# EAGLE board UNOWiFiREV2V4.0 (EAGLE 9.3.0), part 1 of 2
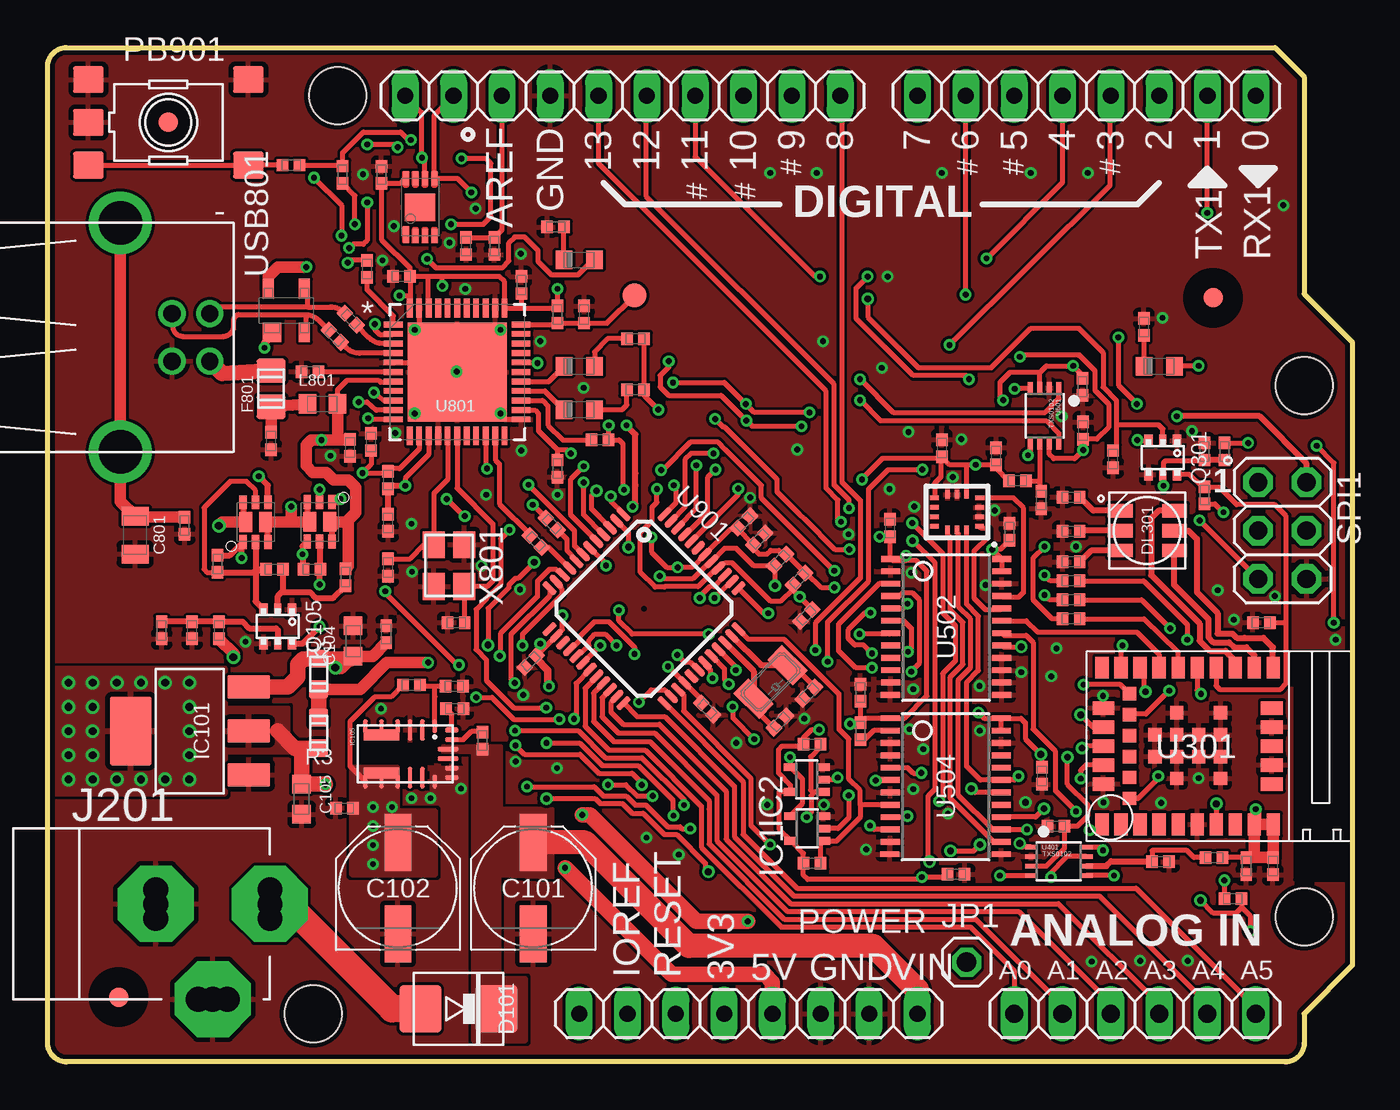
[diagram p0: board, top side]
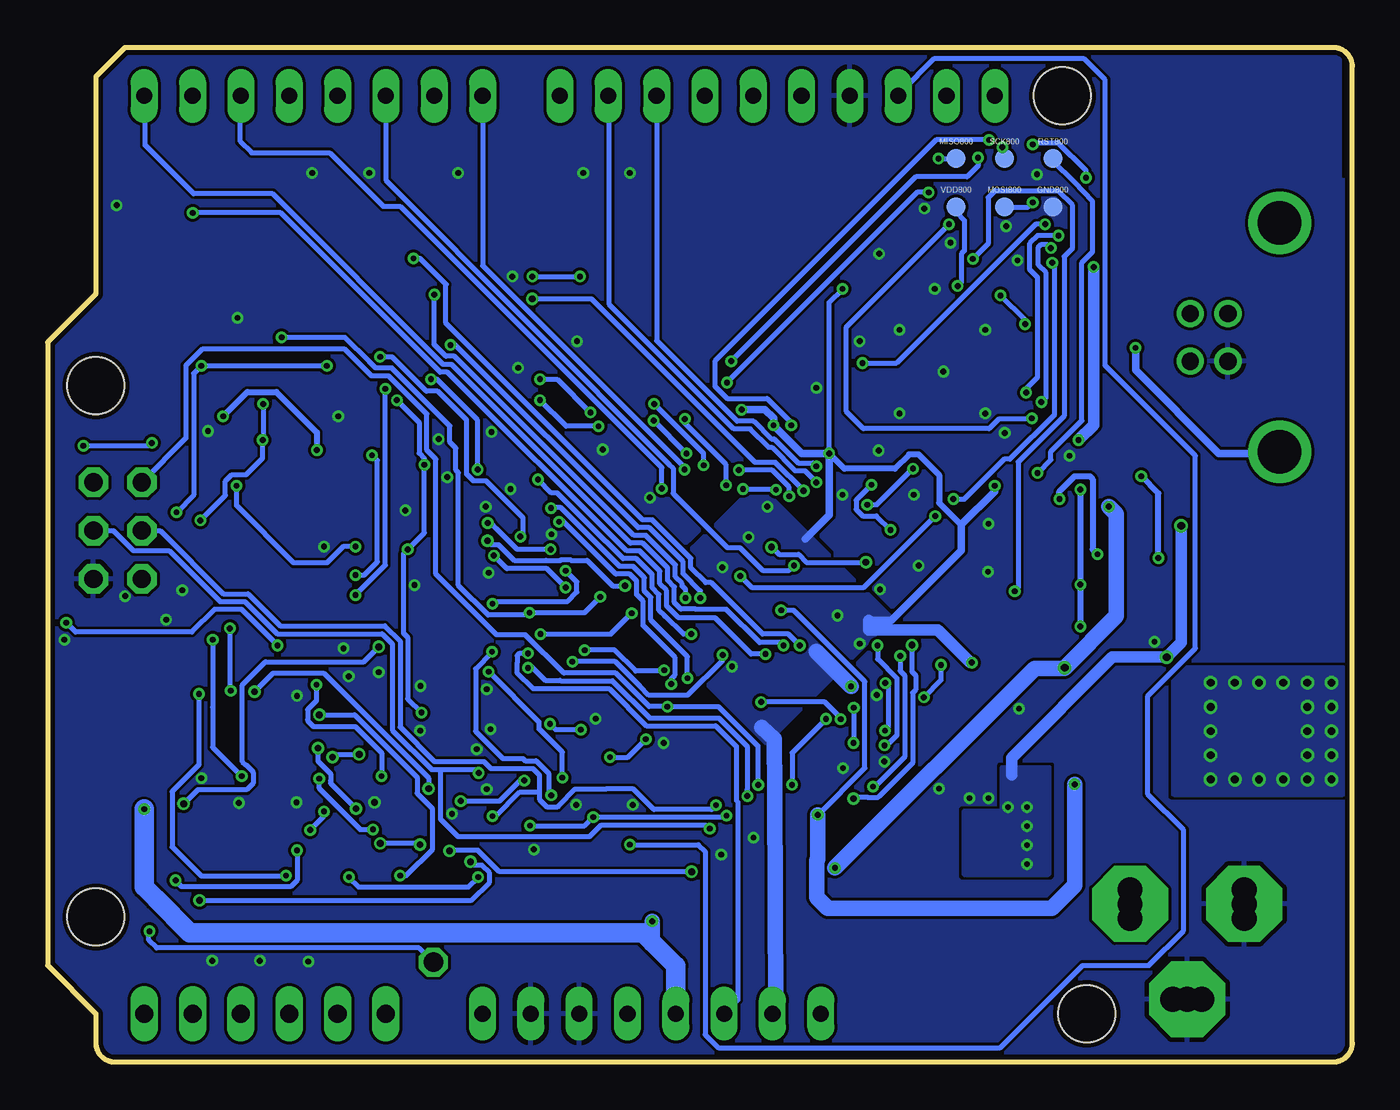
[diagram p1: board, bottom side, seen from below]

Size 68.58 x 53.34 mm. Coordinates in mm from the lower left corner, seen from the top.
Outline: 64.52,53.34 66.04,51.82 66.04,40.39 68.58,37.85 68.58,5.08 66.04,2.54 66.04,1 arc-90 65.04,0 1,0 arc-90 0,1 0,52.34 arc-90 1,53.34 64.52,53.34
Copper layers (1*16): Top 0.035mm / dielectric 1.5mm / Bottom 0.035mm
Design rules "SeeedStudio_2layers": minimum track width 6mil, minimum drill 12mil, track to track 6mil, track to pad 6mil, pad to pad 6mil, via to via 6mil, smd to smd 0mil, copper to edge 10mil, drill to drill 10mil, minimum pad ring 10mil, minimum via ring 6mil, stop-mask expansion 2mil, vias tented up to drill 100mil, thermal gap 10mil
Net classes: 0 default: width 0.006 mm, drill 0.305 mm
Holes 3 mm at 66.04,35.56 66.04,7.62 15.24,50.8 13.97,2.54
tRestrict: 3 lines

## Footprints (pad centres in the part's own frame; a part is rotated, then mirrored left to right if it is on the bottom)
1X06-TH = drill 0.95 pad 1.422 long: 1 -6.35,0; 2 -3.81,0; 3 -1.27,0; 4 1.27,0; 5 3.81,0; 6 6.35,0
0402-1005X55N = smd 0.62 x 0.62: 1 -0.45,0; 2 0.45,0
PANASONIC_D = smd 3 x 1.4: + 2.4,0; - -2.4,0
0603-1608X90N = smd 0.95 x 1: 1 -0.8,0; 2 0.8,0
0805-R2013X50N = smd 0.95 x 1.45: 1 -1,0; 2 1,0
SMB_DO214AA = smd 2.2 x 2.5: A -2,0; C 2,0
SOT190P230X110-4N = smd 1 x 1: 1 -1.15,0.75 | smd 1 x 0.6: 2 -1.15,-0.95; 3 1.15,-0.95; 4 1.15,0.95
RGBLED = smd 1.3 x 0.7: 1 -1.425,1.05; 2 -1.425,0; 3 -1.425,-1.05; 4 1.425,-1.05; 5 1.425,0; 6 1.425,1.05
C0805 = smd 1.25 x 1.5: 1 -0.95,0; 2 0.95,0
FD-1-2 = smd 1.016 x 1.016: P$1 0,0
TP-1.00MM = smd 1 x 1 bottom: X 0,0
SC70-5 = smd 0.4 x 0.7: 1 -0.65,-0.85; 2 0,-0.85; 3 0.65,-0.85; 4 0.65,0.85; 5 -0.65,0.85
SOT223 = smd 2.235 x 1.219: 1 -3.099,2.311; 2 -3.099,0; 3 -3.099,-2.311 | smd 2.2 x 3.6: 4 3.099,0
MPM3610 = smd 0.7 x 0.25: 1 -1.45,1.55; 4 -1.45,-0.4; 5 -1.45,-1.25; 6 -1.45,-2.1; 7 1.45,-2.1; 8 1.45,-1.25; 9 1.45,-0.4; 12 1.45,1.55 | smd 1.1 x 0.25: 2 -1.25,0.9; 3 -1.25,0.25; 10 1.25,0.25; 11 1.25,0.9 | smd 0.25 x 0.7: 13 1.25,2.45; 14 0.75,2.45; 17 -0.75,2.45; 18 -1.25,2.45 | smd 0.25 x 1.1: 15 0.25,2.25; 16 -0.25,2.25 | smd 0.6 x 1.95: 19 -1,-1.25; 20 1,-1.25
1X10 = drill 0.85 pad 1.422 long: 1 -11.43,0; 2 -8.89,0; 3 -6.35,0; 4 -3.81,0; 5 -1.27,0; 6 1.27,0; 7 3.81,0; 8 6.35,0; 9 8.89,0; 10 11.43,0
1X08 = drill 0.85 pad 1.422 long: 1 -8.89,0; 2 -6.35,0; 3 -3.81,0; 4 -1.27,0; 5 1.27,0; 6 3.81,0; 7 6.35,0; 8 8.89,0
POWERSUPPLY_DC-21MM = drill 1.3 pad 4 octagon: +1 -0.076,-6.35; -1 -0.076,-0.356; E1 -5.08,-3.353 | drill 1.3: +2 -0.838,-6.35; +3 0.686,-6.35; -2 -0.838,-0.356; -3 0.686,-0.356; E2 -5.08,-2.591; E3 -5.08,-4.115
1X01 = drill 1.016 octagon: 1 0,0
LEDC1608X80N-AK = smd 0.9 x 0.95: A 0.8,0; C -0.8,0
TS42 = smd 1.6 x 1.4: 1 4.2,-2.25; 2 -4.2,-2.25; 3 4.2,2.25; 4 -4.2,2.25; 5 4.2,0
PWR_SC70 = smd 0.4 x 0.69: D1 -0.65,1.04; D2 0.65,-1.04; G1 0,-1.04; G2 0,1.04; S1 -0.65,-1.04; S2 0.65,1.04 | smd 0.7 x 1: D1' -0.525,0; D2' 0.525,0
SOT363 = smd 0.5 x 0.6: 1 -0.75,-0.9; 3 0.75,-0.9; 4 0.75,0.9; 6 -0.75,0.9 | smd 0.4 x 0.6: 2 0,-0.9; 5 0,0.9
C0603 = smd 0.95 x 1: 1 -0.8,0; 2 0.8,0
2X03 = drill 0.95 pad 1.55 octagon: 1 2.54,1.27; 2 2.54,-1.27; 3 0,1.27; 4 0,-1.27; 5 -2.54,1.27; 6 -2.54,-1.27
TP-1.27MM = smd 1.27 x 1.27 bottom: X 0,0
LGA14L = smd 0.45 x 0.25: 1 -1.175,0.75; 2 -1.175,0.25; 3 -1.175,-0.25; 4 -1.175,-0.75; 8 1.175,-0.75; 9 1.175,-0.25; 10 1.175,0.25; 11 1.175,0.75 | smd 0.25 x 0.45: 5 -0.5,-0.925; 6 0,-0.925; 7 0.5,-0.925; 12 0.5,0.925; 13 0,0.925; 14 -0.5,0.925
NINA-W1X = smd 0.7 x 1.15: 1 4.95,4.125; 2 3.95,4.125; 3 2.95,4.125; 4 1.95,4.125; 5 0.95,4.125; 6 -0.05,4.125; 7 -1.05,4.125; 8 -2.05,4.125; 9 -3.05,4.125; 10 -4.05,4.125; 16 -4.05,-4.125; 17 -3.05,-4.125; 18 -2.05,-4.125; 19 -1.05,-4.125; 20 -0.05,-4.125; 21 0.95,-4.125; 22 1.95,-4.125; 23 2.95,-4.125; 24 3.95,-4.125; 25 4.95,-4.125 | smd 1.15 x 0.7: 11 -3.975,2; 12 -3.975,1; 13 -3.975,0; 14 -3.975,-1; 15 -3.975,-2; 26 4.875,-2; 27 4.875,-1; 28 4.875,0; 29 4.875,1; 30 4.875,2 | smd 0.7 x 0.7: 31 3.5,2.75; 32 3.5,1.65; 33 3.5,0.55; 34 3.5,-0.55; 35 3.5,-1.65; 36 3.5,-2.75; GND@1 -1.28,1.7; GND@2 -1.28,0.55; GND@3 -1.28,-0.6; GND@4 -1.28,-1.75; GND@5 -0.13,0.55; GND@6 -0.13,-0.6; GND@7 1.02,1.7; GND@8 1.02,0.55; GND@9 1.02,-0.6; GND@10 1.02,-1.75; GND@11 2.17,0.55; GND@12 2.17,-0.6
VFSOP-8 = smd 0.25 x 0.65: P$1 -0.75,-1.45; P$2 -0.25,-1.45; P$3 0.25,-1.45; P$4 0.75,-1.45; P$5 0.75,1.45; P$6 0.25,1.45; P$7 -0.25,1.45; P$8 -0.75,1.45
TSSOP24 = smd 0.305 x 0.991: 1 -3.575,-2.918; 2 -2.925,-2.918; 3 -2.275,-2.918; 4 -1.625,-2.918; 5 -0.975,-2.918; 6 -0.325,-2.918; 7 0.325,-2.918; 8 0.975,-2.918; 9 1.625,-2.918; 10 2.275,-2.918; 11 2.925,-2.918; 12 3.575,-2.932; 13 3.575,2.918; 14 2.925,2.918; 15 2.275,2.918; 16 1.625,2.918; 17 0.975,2.918; 18 0.325,2.918; 19 -0.325,2.918; 20 -0.975,2.918; 21 -1.625,2.918; 22 -2.275,2.918; 23 -2.925,2.918; 24 -3.575,2.918
SON50P300X200X60-9N-EP160X140 = smd 0.3 x 0.85: 1 -0.75,-1.45 | smd 0.3 x 0.7: 2 -0.25,-1.525; 3 0.25,-1.525; 4 0.75,-1.525; 5 0.75,1.525; 6 0.25,1.525; 7 -0.25,1.525; 8 -0.75,1.525 | smd 1.6 x 1.4: 9 0,0
QFN50P700X700X100-45N = smd 0.991 x 0.305: 1 -3.353,2.489; 2 -3.353,2.007; 3 -3.353,1.499; 4 -3.353,0.991; 5 -3.353,0.508; 6 -3.353,0; 7 -3.353,-0.508; 8 -3.353,-0.991; 9 -3.353,-1.499; 10 -3.353,-2.007; 11 -3.353,-2.489; 23 3.353,-2.489; 24 3.353,-2.007; 25 3.353,-1.499; 26 3.353,-0.991; 27 3.353,-0.508; 28 3.353,0; 29 3.353,0.508; 30 3.353,0.991; 31 3.353,1.499; 32 3.353,2.007; 33 3.353,2.489 | smd 0.305 x 0.991: 12 -2.489,-3.353; 13 -2.007,-3.353; 14 -1.499,-3.353; 15 -0.991,-3.353; 16 -0.508,-3.353; 17 0,-3.353; 18 0.508,-3.353; 19 0.991,-3.353; 20 1.499,-3.353; 21 2.007,-3.353; 22 2.489,-3.353; 34 2.489,3.353; 35 2.007,3.353; 36 1.499,3.353; 37 0.991,3.353; 38 0.508,3.353; 39 0,3.353; 40 -0.508,3.353; 41 -0.991,3.353; 42 -1.499,3.353; 43 -2.007,3.353; 44 -2.489,3.353 | smd 5.207 x 5.207: 45 0,0
TQFP48 = smd 0.85 x 0.32: 1 -4.275,2.75; 2 -4.275,2.25; 3 -4.275,1.75; 4 -4.275,1.25; 5 -4.275,0.75; 6 -4.275,0.25; 7 -4.275,-0.25; 8 -4.275,-0.75; 9 -4.275,-1.25; 10 -4.275,-1.75; 11 -4.275,-2.25; 12 -4.275,-2.75; 25 4.275,-2.75; 26 4.275,-2.25; 27 4.275,-1.75; 28 4.275,-1.25; 29 4.275,-0.75; 30 4.275,-0.25; 31 4.275,0.25; 32 4.275,0.75; 33 4.275,1.25; 34 4.275,1.75; 35 4.275,2.25; 36 4.275,2.75 | smd 0.32 x 0.85: 13 -2.75,-4.275; 14 -2.25,-4.275; 15 -1.75,-4.275; 16 -1.25,-4.275; 17 -0.75,-4.275; 18 -0.25,-4.275; 19 0.25,-4.275; 20 0.75,-4.275; 21 1.25,-4.275; 22 1.75,-4.275; 23 2.25,-4.275; 24 2.75,-4.275; 37 2.75,4.275; 38 2.25,4.275; 39 1.75,4.275; 40 1.25,4.275; 41 0.75,4.275; 42 0.25,4.275; 43 -0.25,4.275; 44 -0.75,4.275; 45 -1.25,4.275; 46 -1.75,4.275; 47 -2.25,4.275; 48 -2.75,4.275 | smd 0 x 0: EP 0,0
USB-B-H = drill 0.914: D+ 0,1.25; D- 1.981,1.25; GND 0,-1.25; VBUS 1.981,-1.25 | drill 2.286: SHIELD1 -2.718,6.02; SHIELD2 -2.718,-6.02
CRYSTAL-3.2-2.5 = smd 1.4 x 1.15: 1 -1.1,-0.8; 2 1.1,-0.8; 3 1.1,0.8; 4 -1.1,0.8
ABS07 = smd 1.1 x 1.9: 1 -1.25,0; 2 1.25,0

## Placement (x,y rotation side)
AD  Analog  [1X06-TH]  57.15,2.54 0 top
C1  100n  [0402-1005X55N]  22,42.9 270 top
C2  4u7  [0402-1005X55N]  23.48,42.9 270 top
C101  47u  [PANASONIC_D]  25.53,9.14 90 top
C102  47u  [PANASONIC_D]  18.41,9.14 90 top
C103  100n  [0402-1005X55N]  15.6,13.35 180 top
C104  10u  [0603-1608X90N]  16.06,22.13 90 top
C105  10u  [0603-1608X90N]  13.35,13.82 270 top
C106  100n  [0402-1005X55N]  17.8,22.5 90 top
C114  100n  [0402-1005X55N]  6,22.7 270 top
C201  100n  [0402-1005X55N]  47,32.27 90 top
C202  100n  [0402-1005X55N]  49.85,31.85 90 top
C301  100n  [0402-1005X55N]  63,10.3 270 top
C302  100n  [0402-1005X55N]  64.4,10.3 90 top
C303  100n  [0402-1005X55N]  63.8,23.1 180 top
C401  100n  [0402-1005X55N]  58.5,10.53 0 top
C402  100n  [0402-1005X55N]  53,12.4 180 top
C403  100n  [0402-1005X55N]  47.75,9.88 0 top
C503  100n  [0402-1005X55N]  42.73,19.43 90 top
C504  100n  [0402-1005X55N]  44.27,28.07 90 top
C505  100n  [0402-1005X55N]  50.55,27.88 90 top
C506  100n  [0402-1005X55N]  52.27,15.05 270 top
C601  100n  [0402-1005X55N]  52.23,29.55 270 top
C602  100n  [0402-1005X55N]  54.4,35.5 270 top
C603  100n  [0402-1005X55N]  54.42,33.2 90 top
C701  100n  [0402-1005X55N]  17.55,46.65 270 top
C801  4n7  [0805-R2013X50N]  4.6,27.7 270 top
C802  1n  [0402-1005X55N]  11.75,32.65 270 top
C803  1n  [0402-1005X55N]  15.9,32.3 270 top
C804  1u  [0402-1005X55N]  13.8,36.3 180 top
C805  100n  [0402-1005X55N]  17,32.6 90 top
C806  100n  [0402-1005X55N]  17.9,28.35 270 top
C807  100n  [0402-1005X55N]  26.8,31.2 270 top
C808  100n  [0402-1005X55N]  24.9,40.85 270 top
C809  100n  [0402-1005X55N]  18.6,41.3 0 top
C810  12pF  [0402-1005X55N]  21.48,23.1 180 top
C811  12pF  [0402-1005X55N]  17.9,26 90 top
C901  4u7  [0402-1005X55N]  36.6,28.4 45 top
C902  100n  [0402-1005X55N]  37.4,27.5 225 top
C903  100n  [0402-1005X55N]  39.88,23.48 225 top
C904  20p  [0402-1005X55N]  40.02,19.39 225 top
C905  20p  [0402-1005X55N]  38.49,17.87 45 top
C906  100n  [0402-1005X55N]  34.67,18.56 135 top
C907  100n  [0402-1005X55N]  25.39,21.07 45 top
D101  1N4007  [SMB_DO214AA]  21.59,2.79 0 top
D801  PRTR5V  [SOT190P230X110-4N]  12.55,39.51 90 top
DL301  RGB  [RGBLED]  57.8,27.94 180 top
F801  [C0805]  11.75,35.4 90 top
FD1  DNP  [FD-1-2]  3.73,3.41 0 top
FD2  DNP  [FD-1-2]  61.26,40.18 0 top
FD3  DNP  [FD-1-2]  6.35,49.4 0 top
FRAME1  DNP  [FRAME]  0,0 0 top
FRAME101  DNP  [FRAME]  0,0 0 top
FRAME201  DNP  [FRAME]  0,0 0 top
FRAME301  DNP  [FRAME]  0,0 0 top
FRAME401  DNP  [FRAME]  0,0 0 top
FRAME501  DNP  [FRAME]  0,0 0 top
FRAME601  DNP  [FRAME]  0,0 0 top
FRAME701  DNP  [FRAME]  0,0 0 top
FRAME801  DNP  [FRAME]  0,0 0 top
FRAME901  DNP  [FRAME]  0,0 0 top
GND800  DNP  [TP-1.00MM]  15.75,44.96 0 top
IC1  74LVC1G125DCKR  [SC70-5]  39.92,12.28 90 top
IC2  74LVC1G125DCKR  [SC70-5]  39.9,14.85 90 top
IC101  -  [SOT223]  7.47,17.4 180 top
IC105  MPM3610  [MPM3610]  18.8,16.2 270 top
IOH  Digital  [1X10]  30.23,50.8 180 top
IOL  Digital  [1X08]  54.61,50.8 180 top
J201  -  [POWERSUPPLY_DC-21MM]  5.33,8.38 90 top
JP1  [1X01]  48.3,5.25 0 top
L801  BLM18PG471  [0603-1608X90N]  14.45,34.6 0 top
LRX800  YELLOW  [LEDC1608X80N-AK]  27.94,34.29 0 top
LTX800  YELLOW  [LEDC1608X80N-AK]  27.94,36.58 0 top
MISO800  DNP  [TP-1.00MM]  20.83,47.5 0 top
MOSI800  DNP  [TP-1.00MM]  18.29,44.96 0 top
ON100  GREEN  [LEDC1608X80N-AK]  58.42,36.58 0 top
PB901  -  [TS42]  6.35,49.4 180 top
POWER  Power  [1X08]  36.83,2.54 0 top
Q101  DMP2160  [PWR_SC70]  14.3,28.4 180 top
Q102  DMP2160  [PWR_SC70]  10.93,28.39 0 top
Q105  BSS138PS  [SOT363]  12.1,22.9 180 top
Q301  BSS138PS  [SOT363]  58.62,31.78 180 top
R1  1k  [0402-1005X55N]  26.7,43.9 180 top
R2  0R  [C0603]  14.25,20.4 270 top
R3  DNP  [C0603]  14.25,17.3 90 top
R4  0R  [0402-1005X55N]  62.3,8.6 0 top
R5  100k  [0402-1005X55N]  40.17,16.7 180 top
R11  100k  [0402-1005X55N]  40.17,10.45 180 top
R101  330R  [0402-1005X55N]  57.62,38.65 90 top
R102  100k  [0402-1005X55N]  19.12,19.82 180 top
R123  100k  [0402-1005X55N]  9,22.7 270 top
R124  100k  [0402-1005X55N]  7.6,22.7 90 top
R125  100k  [0402-1005X55N]  15.66,25.49 90 top
R126  330R  [0402-1005X55N]  11.92,25.9 0 top
R127  10k  [0402-1005X55N]  13.9,25.9 180 top
R128  10k  [0402-1005X55N]  8.92,26.19 90 top
R129  19k1  [0402-1005X55N]  21.38,19.75 180 top
R130  100k  [0402-1005X55N]  22.85,16.9 90 top
R131  53k6  [0402-1005X55N]  21.4,18.57 180 top
R301  100k  [0402-1005X55N]  60.8,29.8 270 top
R302  100k  [0402-1005X55N]  56,31.7 270 top
R303  0R  [0402-1005X55N]  53.8,24.3 180 top
R304  0R  [0402-1005X55N]  53.8,25.3 180 top
R305  330R  [0402-1005X55N]  53.8,27.9 0 top
R306  330R  [0402-1005X55N]  53.8,26.3 0 top
R307  330R  [0402-1005X55N]  53.8,29.7 0 top
R308  100k  [0402-1005X55N]  60.8,32.1 90 top
R309  DNP  [0402-1005X55N]  61.85,32.1 90 top
R310  0R  [0402-1005X55N]  53.8,23.3 0 top
R405  100k  [0402-1005X55N]  61.3,10.75 0 top
R504  100k  [0402-1005X55N]  42.73,17.4 90 top
R605  100k  [0402-1005X55N]  50.98,30.55 180 top
R801  1M  [0402-1005X55N]  7.2,28.2 90 top
R802  330R  [0402-1005X55N]  16.8,41.7 90 top
R803  100k  [0402-1005X55N]  17.9,30.6 270 top
R804  1k  [0402-1005X55N]  26.5,28.29 135 top
R805  1k  [0402-1005X55N]  25.66,27.37 135 top
R806  0R  [0402-1005X55N]  29.03,32.71 0 top
R807  1k  [0402-1005X55N]  30.9,35.35 0 top
R808  1k  [0402-1005X55N]  30.9,38.02 0 top
R809  100k  [0402-1005X55N]  26.8,39.3 90 top
R810  DNP  [0402-1005X55N]  28.2,39.3 270 top
R811  22R  [0402-1005X55N]  15.93,39.06 135 top
R812  22R  [0402-1005X55N]  15.09,38.16 135 top
R901  DNP  [0402-1005X55N]  38.5,26.4 45 top
R902  100k  [0402-1005X55N]  39.5,25.4 45 top
R903  330R  [0402-1005X55N]  15.5,46.65 270 top
R904  39R  [0402-1005X55N]  12.8,47.16 180 top
RST800  DNP  [TP-1.00MM]  15.75,47.5 0 top
SCK800  DNP  [TP-1.00MM]  18.29,47.5 0 top
SPI1  -  [2X03]  64.9,27.94 90 top
TP801  DNP  [TP-1.27MM]  30.85,40.3 0 bottom
U201  LSM6DSMTR  [LGA14L]  47.8,28.91 180 top
U301  NINA-W132  [NINA-W1X]  60.37,16.61 180 top
U401  TXS0102  [VFSOP-8]  53.15,10.55 270 top
U502  MC74LVX4245  [TSSOP24]  47.23,22.88 270 top
U504  MC74LVX4245  [TSSOP24]  47.2,14.5 270 top
U601  TXS0102  [VFSOP-8]  52.4,33.98 180 top
U701  ECC608  [SON50P300X200X60-9N-EP160X140]  19.58,44.94 0 top
U801  ATMEGA32U4RC  [QFN50P700X700X100-45N]  21.53,36.28 0 top
U901  ATMEGA4809  [TQFP48]  31.35,23.83 315 top
USB801  -  [USB-B-H]  6.54,38.1 0 top
USR  YELLOW  [LEDC1608X80N-AK]  27.94,42.16 0 top
VDD800  DNP  [TP-1.00MM]  20.83,44.96 0 top
X801  16MHz  [CRYSTAL-3.2-2.5]  21.1,26.1 270 top
Y901  32768Hz  [ABS07]  37.99,19.98 45 top

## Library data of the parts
AD = Arduino-connectors; CODE-ARDUINO: 3649; DATASHEET: -; DISTRIBUTOR-LINK: -; DISTRIBUTOR-PN: -; MANUFACTURER: -; MANUFACTURER-PN: FH254-106DF085149V
C1 C103 C106 C114 C201 C202 C301-C303 C401-C403 C503-C506 C601-C603 C701 C805-C809 C902 C903 C906 C907 = Arduino-rcl; CODE-ARDUINO: 0132; DATASHEET: http://www.tdk.com/pdf/TDKMLCCCapRange.pdf; DISTRIBUTOR-LINK: http://www.digikey.com/product-detail/en/tdk-corporation/C1005X5R1H104K050BB/445-5942-1-ND/2443982; DISTRIBUTOR-PN: 445-5942-1-ND; MANUFACTURER: TDK; MANUFACTURER-PN: C1005X5R1H104K050BB; NOTE: -
C2 C901 = Arduino-rcl; CODE-ARDUINO: 0833; DATASHEET: http://search.murata.co.jp/Ceramy/image/img/A01X/partnumbering_e_01.pdf; DISTRIBUTOR-LINK: http://www.digikey.com/product-detail/en/murata-electronics-north-america/GRM155R60J475ME47D/490-5915-1-ND/3719860; DISTRIBUTOR-PN: 490-5915-1-ND; MANUFACTURER: Murata; MANUFACTURER-PN: GRM155R60J475ME47D; NOTE: -
C101 C102 = Arduino-rcl; CODE-ARDUINO: 0113; DATASHEET: https://industrial.panasonic.com/cdbs/www-data/pdf/RDE0000/DME0000COL90.pdf; DISTRIBUTOR-LINK: https://www.digikey.com/product-detail/en/panasonic-electronic-components/EEE-1EA470WP/PCE3908CT-ND/766284; DISTRIBUTOR-PN: PCE3908CT-ND; MANUFACTURER: Panasonic; MANUFACTURER-PN: EEE-1EA470WP; PN-ALTERNATIVE1: TS13C01E470MET000R
C104 C105 = Arduino-rcl; CODE-ARDUINO: 2213; DATASHEET: http://www.murata.com/~/media/webrenewal/support/library/catalog/products/capacitor/mlcc/c02e.pdf; DISTRIBUTOR-LINK: http://www.digikey.com/product-search/en?keywords=490-10728-1-ND; DISTRIBUTOR-PN: 490-10728-1-ND; MANUFACTURER: Murata; MANUFACTURER-PN: GRM188R61C106KAALD; NOTE: -
C801 = Arduino-rcl; CODE-ARDUINO: 0689; DATASHEET: http://www.kemet.com/Lists/ProductCatalog/Attachments/40/KEM_C1010_X7R_HV_SMD.pdf; DISTRIBUTOR-LINK: www.kemet.com/docfinder?Partnumber=C0805C472KDRACTU; DISTRIBUTOR-PN: 399-6738-1-ND; MANUFACTURER: Kemet; MANUFACTURER-PN: C0805C472KDRACTU; NOTE: -
C802 C803 = Arduino-rcl; CODE-ARDUINO: 2321; DATASHEET: http://www.samsungsem.com/kr/support/product-search/mlcc/__icsFiles/afieldfile/2016/08/18/S_CL05B102KB5NNNC.pdf; DISTRIBUTOR-LINK: http://www.digikey.com/product-detail/en/samsung-electro-mechanics-america-inc/CL05B102KB5NNNC/1276-1032-1-ND/3889118; DISTRIBUTOR-PN: 1276-1032-1-ND; MANUFACTURER: Samsung; MANUFACTURER-PN: CL05B102KB5NNNC; NOTE: -
C804 = Arduino-rcl; CODE-ARDUINO: 0133; DATASHEET: http://search.murata.co.jp/Ceramy/image/img/A01X/partnumbering_e_01.pdf; DISTRIBUTOR-LINK: http://www.digikey.com/product-detail/en/murata-electronics-north-america/GRM155R61E105KA12D/490-10017-1-ND/5026367; DISTRIBUTOR-PN: 490-10017-1-ND; MANUFACTURER: Murata; MANUFACTURER-PN: GRM155R61E105KA12D; NOTE: -
C810 C811 = Arduino-rcl; CODE-ARDUINO: A5006; DATASHEET: http://search.murata.co.jp/Ceramy/image/img/A01X/partnumbering_e_01.pdf; DISTRIBUTOR-LINK: https://www.digikey.com/product-detail/en/murata-electronics-north-america/GJM1555C1H120GB01D/490-8078-1-ND/4380364; DISTRIBUTOR-PN: 490-8078-1-ND; MANUFACTURER: Murata; MANUFACTURER-PN: GJM1555C1H120GB01D; NOTE: -
C904 C905 = Arduino-rcl; CODE-ARDUINO: 2188; DATASHEET: http://www.kemet.com/docfinder?Partnumber=CBR04C200J5GAC; DISTRIBUTOR-LINK: http://www.digikey.com/product-detail/en/kemet/CBR04C200J5GAC/399-6173-1-ND/2732143; DISTRIBUTOR-PN: 399-6173-1-ND; MANUFACTURER: Kemet; MANUFACTURER-PN: CBR04C200J5GAC; NOTE: -
D101 = Arduino-diodes; CODE-ARDUINO: 0020; DATASHEET: www.comchiptech.com/cms/UserFiles/CGRA4001-G%20Thru.%20CGRA4007-HF%20RevD.pdf; DISTRIBUTOR-LINK: https://www.digikey.com/product-detail/en/comchip-technology/CGRA4007-G/641-1018-1-ND/1121140; DISTRIBUTOR-PN: 641-1018-1-ND; MANUFACTURER: Comchip; MANUFACTURER-PN: CGRA4007-G; PN-ALTERNATIVE1: 1N4007SMA
D801 = Arduino-diodes; CODE-ARDUINO: 2209; DATASHEET: http://www.nxp.com/documents/data_sheet/PRTR5V0U2X.pdf; DISTRIBUTOR-LINK: http://www.digikey.com/product-detail/en/nxp-semiconductors/PRTR5V0U2X,215/568-4140-1-ND/1589981; DISTRIBUTOR-PN: 568-4140-1-ND; MANUFACTURER: NXP; MANUFACTURER-PN: PRTR5V0U2X,215
DL301 = Arduino-diodes; CODE-ARDUINO: 2211; DATASHEET: http://www.osram-os.com/Graphics/XPic9/00134830_0.pdf; DISTRIBUTOR-LINK: https://www.digikey.com/product-detail/en/osram-opto-semiconductors-inc/LTRBGFSF-ABCB-QKYO-Z/475-2899-1-ND/2415091; DISTRIBUTOR-PN: 475-2899-1-ND; MANUFACTURER: OSRAM Opto Semiconductors Inc.; MANUFACTURER-PN: LTRBGFSF-ABCB-QKYO-Z
F801 = Arduino-rcl; CODE-ARDUINO: 0002; DATASHEET: https://www.bourns.com/docs/Product-Datasheets/mfmsmf.pdf; DISTRIBUTOR-LINK: https://www.digikey.it/product-detail/en/bourns-inc/MF-MSMF050-2/MF-MSMF050-2CT-ND/662842; DISTRIBUTOR-PN: MF-MSMF050-2CT-ND; MANUFACTURER: Bourns; MANUFACTURER-PN: MF-MSMF050-2
FD1-FD3 GND800 MISO800 MOSI800 RST800 SCK800 TP801 VDD800 = Arduino-utility; CODE-ARDUINO: DNP; DATASHEET: DNP; DISTRIBUTOR-LINK: DNP; DISTRIBUTOR-PN: DNP; MANUFACTURER: DNP; MANUFACTURER-PN: DNP
FRAME1 FRAME101 FRAME201 FRAME301 FRAME401 FRAME501 FRAME601 FRAME701 FRAME801 FRAME901 = Arduino-utility; CODE-ARDUINO: DNP; DATASHEET: DNP; DISTRIBUTOR-LINK: DNP; DISTRIBUTOR-PN: DNP; MANUFACTURER: DNP; MANUFACTURER-PN: DNP; NOTE: DNP
IC1 IC2 = Arduino-ICs; CODE-ARDUINO: 0040; DATASHEET: http://www.ti.com/lit/ds/symlink/sn74lvc1g125.pdf; DISTRIBUTOR-LINK: https://www.digikey.com/product-detail/en/texas-instruments/SN74LVC1G125DCKR/296-11604-1-ND/385743; DISTRIBUTOR-PN: 296-11604-1-ND; MANUFACTURER: Texas Instruments; MANUFACTURER-PN: SN74LVC1G125DCKR; NOTE: NO
IC101 = Arduino-ICs; CODE-ARDUINO: 0045; DATASHEET: https://media.digikey.com/pdf/Data%20Sheets/NXP%20PDFs/NX1117C(E).pdf; DISTRIBUTOR-LINK: https://www.digikey.com/product-detail/en/nxp-usa-inc/NX1117CE33Z,115/568-8443-1-ND/2765160; DISTRIBUTOR-PN: 568-8443-1-ND; MANUFACTURER: NXP; MANUFACTURER-PN: NX1117CE33Z,115; NOTE: NO
IC105 = Arduino-ICs; CODE-ARDUINO: 2093; DATASHEET: https://www.monolithicpower.com/pub/media/document/MPM3610_r1.01.pdf; DISTRIBUTOR-LINK: https://www.digikey.com/product-detail/en/monolithic-power-systems-inc/MPM3610AGQV-P/1589-1249-1-ND/5298336; DISTRIBUTOR-PN: 1589-1249-1-ND; MANUFACTURER: MPS; MANUFACTURER-PN: MPM3610AGQV-P; RESTRICTIONS: NO
IOH = Arduino-connectors; CODE-ARDUINO: 3648; DATASHEET: -; DISTRIBUTOR-LINK: -; DISTRIBUTOR-PN: -; MANUFACTURER: -; MANUFACTURER-PN: FH254-110DF085149V
IOL = Arduino-connectors; CODE-ARDUINO: 3648; DATASHEET: -; DISTRIBUTOR-LINK: -; DISTRIBUTOR-PN: -; MANUFACTURER: -; MANUFACTURER-PN: FH254-108DF085149V
J201 = Arduino-connectors; CODE-ARDUINO: 0018; DATASHEET: http://www.mouser.com/ds/2/253/KC-301287-195995.pdf; DISTRIBUTOR-LINK: https://www.mouser.it/ProductDetail/Kobiconn/163-179PH-EX/?qs=Xb8IjHhkxj5l2UOaIqcGCw==; DISTRIBUTOR-PN: 163-179PH-EX; MANUFACTURER: Kobiconn; MANUFACTURER-PN: 163-179PH-EX
JP1 = pinhead
L801 = Arduino-rcl; CODE-ARDUINO: 2217; DATASHEET: http://search.murata.co.jp/Ceramy/image/img/PDF/ENG/L0110S0100BLM18P.pdf; DISTRIBUTOR-LINK: http://www.digikey.com/product-detail/en/murata-electronics-north-america/BLM18PG471SN1D/490-5223-1-ND/1948399; DISTRIBUTOR-PN: 490-5223-1-ND; MANUFACTURER: Murata; MANUFACTURER-PN: BLM18PG471SN1D; NOTE: -
LRX800 LTX800 USR = Arduino-diodes; CODE-ARDUINO: 2243; DATASHEET: http://media.digikey.com/pdf/Data%20Sheets/Avago%20PDFs/HSMz-Czzz.pdf; DISTRIBUTOR-LINK: http://www.digikey.com/product-detail/en/broadcom-limited/HSMY-C190/516-1424-1-ND/637748; DISTRIBUTOR-PN: 516-1424-1-ND; MANUFACTURER: Avago; MANUFACTURER-PN: HSMY-C190
ON100 = Arduino-diodes; CODE-ARDUINO: 2204; DATASHEET: http://media.digikey.com/pdf/Data%20Sheets/Avago%20PDFs/HSMz-Czzz.pdf; DISTRIBUTOR-LINK: http://www.digikey.com/product-detail/en/broadcom-limited/HSMG-C190/516-1425-1-ND/637749; DISTRIBUTOR-PN: 516-1425-1-ND; MANUFACTURER: Avago; MANUFACTURER-PN: HSMG-C190
PB901 = Arduino-pushbuttons; CODE-ARDUINO: 0946; DATASHEET: http://www.mouser.com/ds/2/418/NG_CD_1571636_C1-122399.pdf; DISTRIBUTOR-LINK: https://www.mouser.it/ProductDetail/TE-Connectivity/1571636-3/?qs=%2fha2pyFaduiys%2fNUBzym%252bcoSb9tuK3Sjuv54qjf0hQ0%3d; DISTRIBUTOR-PN: 506-1571636-3; MANUFACTURER: TE; MANUFACTURER-PN: 1571636-3; PN-ALTERNATIVE1: TS42031-160WWS027260
POWER = Arduino-connectors; CODE-ARDUINO: 3649; DATASHEET: -; DISTRIBUTOR-LINK: -; DISTRIBUTOR-PN: -; MANUFACTURER: -; MANUFACTURER-PN: FH254-108DF085149V
Q101 Q102 = Arduino-transistors; CODE-ARDUINO: 2324; DATASHEET: http://www.diodes.com/_files/datasheets/ds31643.pdf; DISTRIBUTOR-LINK: http://www.digikey.com/product-detail/en/diodes-incorporated/DMP2160UFDB-7/DMP2160UFDB-7DI-ND/4249940; DISTRIBUTOR-PN: DMP2160UFDB-7DI-ND; MANUFACTURER: Diodes Inc; MANUFACTURER-PN: DMP2160UFDB-7
Q105 Q301 = Arduino-transistors; CODE-ARDUINO: 2323; DATASHEET: https://assets.nexperia.com/documents/data-sheet/BSS138PS.pdf; DISTRIBUTOR-LINK: http://www.digikey.com/product-detail/en/nxp-semiconductors/BSS138PS,115/568-8393-1-ND/2763927; DISTRIBUTOR-PN: 568-8393-1-ND; MANUFACTURER: NXP; MANUFACTURER-PN: BSS138PS,115
R1 R804 R805 R807 R808 = Arduino-rcl; CODE-ARDUINO: 0140; DATASHEET: www.yageo.com.tw/exep/pages/download/literatures/PYu-R_INT-thick_7.pdf; DISTRIBUTOR-LINK: http://www.digikey.com/product-detail/en/yageo/RC0402FR-071KL/311-1.00KLRCT-ND/729460; DISTRIBUTOR-PN: 311-1.00KLRCT-ND; MANUFACTURER: Yageo; MANUFACTURER-PN: RC0402FR-071KL; NOTE: NO
R2 = Arduino-rcl; CODE-ARDUINO: 0233; DATASHEET: http://www.yageo.com/exep/pages/download/literatures/PYu-R_Marking_2.pdf; DISTRIBUTOR-LINK: https://www.digikey.com/product-detail/en/yageo/RC0603JR-070RL/311-0.0GRCT-ND/729622; DISTRIBUTOR-PN: 311-0.0GRCT-ND; MANUFACTURER: Yageo; MANUFACTURER-PN: RC0603JR-070RL; NOTE: NO
R3 = Arduino-rcl; CODE-ARDUINO: DNP; DATASHEET: DNP; DISTRIBUTOR-LINK: DNP; DISTRIBUTOR-PN: DNP; MANUFACTURER: DNP; MANUFACTURER-PN: DNP; NOTE: DNP
R4 R303 R304 R310 R806 = Arduino-rcl; CODE-ARDUINO: 0039; DATASHEET: www.yageo.com.tw/exep/pages/download/literatures/PYu-R_INT-thick_7.pdf; DISTRIBUTOR-LINK: http://www.digikey.com/product-detail/en/yageo/RC0402FR-070RL/311-0.0LRCT-ND/2827888; DISTRIBUTOR-PN: 311-0.0LRCT-ND; MANUFACTURER: Yageo; MANUFACTURER-PN: RC0402FR-070RL; NOTE: NO
R5 R11 R102 R123-R125 R130 R301 R302 R308 R405 R504 R605 R803 R809 R902 = Arduino-rcl; CODE-ARDUINO: 0134; DATASHEET: www.yageo.com.tw/exep/pages/download/literatures/PYu-R_INT-thick_7.pdf; DISTRIBUTOR-LINK: http://www.digikey.com/product-detail/en/yageo/RC0402FR-07100KL/311-100KLRCT-ND/729473; DISTRIBUTOR-PN: 311-100KLRCT-ND; MANUFACTURER: Yageo; MANUFACTURER-PN: RC0402FR-07100KL; NOTE: NO
R101 R126 R305-R307 R802 R903 = Arduino-rcl; CODE-ARDUINO: 2229; DATASHEET: www.yageo.com.tw/exep/pages/download/literatures/PYu-R_INT-thick_7.pdf; DISTRIBUTOR-LINK: http://www.digikey.com/product-detail/en/yageo/RC0402FR-07330RL/311-330LRCT-ND/729541; DISTRIBUTOR-PN: 311-330LRCT-ND; MANUFACTURER: Yageo; MANUFACTURER-PN: RC0402FR-07330RL; NOTE: NO
R127 R128 = Arduino-rcl; CODE-ARDUINO: 0136; DATASHEET: www.yageo.com.tw/exep/pages/download/literatures/PYu-R_INT-thick_7.pdf; DISTRIBUTOR-LINK: http://www.digikey.com/product-detail/en/yageo/RC0402FR-0710KL/311-10.0KLRCT-ND/729470; DISTRIBUTOR-PN: 311-10.0KLRCT-ND; MANUFACTURER: Yageo; MANUFACTURER-PN: RC0402FR-0710KL; NOTE: NO
R129 = Arduino-rcl; CODE-ARDUINO: A5369; DATASHEET: www.yageo.com.tw/exep/pages/download/literatures/PYu-R_INT-thick_7.pdf; DISTRIBUTOR-LINK: https://www.digikey.com/product-detail/en/yageo/RC0402FR-0719K1L/311-19.1KLRCT-ND/729499; DISTRIBUTOR-PN: 311-19.1KLRCT-ND; MANUFACTURER: Yageo; MANUFACTURER-PN: RC0402FR-0719K1L; NOTE: 1% ONLY
R131 = Arduino-rcl; CODE-ARDUINO: A5313; DATASHEET: www.yageo.com.tw/exep/pages/download/literatures/PYu-R_INT-thick_7.pdf; DISTRIBUTOR-LINK: https://www.digikey.com/product-detail/en/yageo/RC0402FR-0753K6L/311-53.6KLRCT-ND/729581; DISTRIBUTOR-PN: 311-53.6KLRCT-ND; MANUFACTURER: Yageo; MANUFACTURER-PN: RC0402FR-0753K6L; NOTE: 1% ONLY
R309 R810 R901 = Arduino-rcl; CODE-ARDUINO: DNP; DATASHEET: DNP; DISTRIBUTOR-LINK: DNP; DISTRIBUTOR-PN: DNP; MANUFACTURER: DNP; MANUFACTURER-PN: DNP; NOTE: NO
R801 = Arduino-rcl; CODE-ARDUINO: 0139; DATASHEET: www.yageo.com.tw/exep/pages/download/literatures/PYu-R_INT-thick_7.pdf; DISTRIBUTOR-LINK: http://www.digikey.com/product-detail/en/yageo/RC0402JR-07330RL/311-330JRCT-ND/729412; DISTRIBUTOR-PN: 311-330JRCT-ND; MANUFACTURER: Yageo; MANUFACTURER-PN: RC0402JR-07330RL; NOTE: NO
R811 R812 = Arduino-rcl; CODE-ARDUINO: 0468; DATASHEET: www.yageo.com.tw/exep/pages/download/literatures/PYu-R_INT-thick_7.pdf; DISTRIBUTOR-LINK: http://www.digikey.com/products/en?keywords=311-22.0LRCT-ND; DISTRIBUTOR-PN: 311-22.0LRCT-ND; MANUFACTURER: Yageo; MANUFACTURER-PN: RC0402FR-0722RL; NOTE: NO
R904 = Arduino-rcl; CODE-ARDUINO: 0138; DATASHEET: www.yageo.com.tw/exep/pages/download/literatures/PYu-R_INT-thick_7.pdf; DISTRIBUTOR-LINK: http://www.digikey.com/product-detail/en/yageo/RC0402FR-0739RL/311-39.0LRCT-ND/729549; DISTRIBUTOR-PN: 311-39.0LRCT-ND; MANUFACTURER: Yageo; MANUFACTURER-PN: RC0402FR-0739RL; NOTE: NO
SPI1 = Arduino-connectors; CODE-ARDUINO: 0114; DATASHEET: -; DISTRIBUTOR-LINK: https://www.digikey.com/product-detail/en/samtec-inc/TSW-103-25-S-D/TSW-103-25-S-D-ND/7863771; DISTRIBUTOR-PN: TSW-103-25-S-D-ND; MANUFACTURER: Samtec; MANUFACTURER-PN: TSW-103-25-S-D
U201 = Arduino-Sensors; CODE-ARDUINO: 2326; DATASHEET: http://www.st.com/content/ccc/resource/technical/document/datasheet/76/27/cf/88/c5/03/42/6b/DM00218116.pdf/files/DM00218116.pdf/jcr:content/translations/en.DM00218116.pdf; DISTRIBUTOR-LINK: https://www.digikey.com/product-detail/en/stmicroelectronics/LSM6DSMTR/497-16696-1-ND/6192778; DISTRIBUTOR-PN: 497-16696-1-ND; MANUFACTURER: ST; MANUFACTURER-PN: LSM6DSMTR
U301 = Arduino-ucs&SoCs; CODE-ARDUINO: 2329; DATASHEET: https://www.u-blox.com/sites/default/files/NINA-W1_DataSheet_%28UBX-17006694%29.pdf; DISTRIBUTOR-LINK: https://www.digikey.com/product-detail/en/u-blox-america-inc/NINA-W132/672-1072-1-ND/7931822; DISTRIBUTOR-PN: 672-1072-1-ND; MANUFACTURER: Ublocks; MANUFACTURER-PN: NINA-W132
U401 U601 = Arduino-ICs; CODE-ARDUINO: A5332; DATASHEET: http://www.ti.com/lit/ds/symlink/txs0102.pdf; DISTRIBUTOR-LINK: http://www.digikey.com/product-detail/en/texas-instruments/TXS0102DCURG4/296-41875-1-ND/5224578; DISTRIBUTOR-PN: 296-41875-1-ND; MANUFACTURER: Texas Instruments; MANUFACTURER-PN: TXS0102DCURG4; NOTE: NO
U502 U504 = Arduino-ICs; CODE-ARDUINO: A5327; DATASHEET: http://www.onsemi.com/pub/Collateral/MC74LVX4245-D.PDF; DISTRIBUTOR-LINK: https://www.digikey.com/product-detail/en/on-semiconductor/MC74LVX4245DTR2G/MC74LVX4245DTR2GOSCT-ND/2120954; DISTRIBUTOR-PN: MC74LVX4245DTR2GOSCT-ND; MANUFACTURER: ON Semiconductor; MANUFACTURER-PN: MC74LVX4245DTR2G; NOTE: NO
U701 = Arduino-ICs; CODE-ARDUINO: A5007; DATASHEET: http://ww1.microchip.com/downloads/en/DeviceDoc/40001977A.pdf; DISTRIBUTOR-LINK: https://www.digikey.com/product-detail/en/microchip-technology/ATECC608A-MAHDA-T/ATECC608A-MAHDA-TCT-ND/7928236; DISTRIBUTOR-PN: ATECC608A-MAHDA-TCT-ND; MANUFACTURER: Microchip; MANUFACTURER-PN: ATECC608A-MAHDA-T; NOTE: NO
U801 = Arduino-ucs&SoCs; CODE-ARDUINO: 0159; DATASHEET: http://ww1.microchip.com/downloads/en/DeviceDoc/Atmel-7766-8-bit-AVR-ATmega16U4-32U4_Datasheet.pdf; DISTRIBUTOR-LINK: https://www.digikey.com/product-detail/en/microchip-technology/ATMEGA32U4RC-MU/ATMEGA32U4RC-MU-ND/2507984; DISTRIBUTOR-PN: ATMEGA32U4RC-MU-ND; MANUFACTURER: Microchip; MANUFACTURER-PN: ATMEGA32U4RC-MU
U901 = Arduino-ucs&SoCs; CODE-ARDUINO: 2322; DATASHEET: http://ww1.microchip.com/downloads/en/DeviceDoc/40002016A.pdf; DISTRIBUTOR-LINK: https://www.digikey.com/product-detail/en/microchip-technology/ATMEGA4809-AFR/ATMEGA4809-AFRCT-ND/8540756; DISTRIBUTOR-PN: ATMEGA4809-AFRCT-ND; MANUFACTURER: Microchip; MANUFACTURER-PN: ATMEGA4809-AFR
USB801 = Arduino-connectors; CODE-ARDUINO: 0056; DATASHEET: http://cnctech.us/pdfs/1001-003-02000.pdf; DISTRIBUTOR-LINK: https://www.digikey.com/products/it?keywords=1001-003-02000; DISTRIBUTOR-PN: 1175-1002-ND; MANUFACTURER: CNC Tech; MANUFACTURER-PN: 1001-003-02000; PN-ALTERNATIVE1: USB-B-S-RA-WT-SPCC
X801 = Arduino-crystals; CODE-ARDUINO: 0395; DATASHEET: https://www.ecsxtal.com/store/pdf/ECX-33Q.pdf; DISTRIBUTOR-LINK: https://www.digikey.com/product-detail/en/ecs-inc/ECS-160-12-33Q-JES-TR/XC2147CT-ND/6050976; DISTRIBUTOR-PN: XC2147CT-ND; MANUFACTURER: ECS; MANUFACTURER-PN: ECS-160-12-33Q-JES-TR
Y901 = Arduino-crystals; CODE-ARDUINO: 0213; DATASHEET: http://www.abracon.com/Resonators/ABS07.pdf; DISTRIBUTOR-LINK: http://www.digikey.com/product-detail/en/abracon-llc/ABS07-32.768KHZ-T/535-9542-1-ND/1237009; DISTRIBUTOR-PN: 535-9542-1-ND; MANUFACTURER: Abracon LLC; MANUFACTURER-PN: ABS07-32.768KHZ-T

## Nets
2XTRANSLATOR1:N$1: C601.1 R605.1 U601.P$6
2XTRANSLATOR2:N$1: C401.1 R405.1 U401.P$6
16XTRANSLATOR1:N$1: R504.1 U504.2
+3V3: C105.1 C201.1 C202.1 C301.1 C302.2 C402.1 C505.1 C506.1 C602.1 IC101.2 IC101.4 ON100.A POWER.4 R3.1 R301.2 R405.2 R605.2 U201.5 U201.8 U301.9 U301.10 U401.P$3 U502.23 U502.24 U504.23 U504.24 U601.P$3
+5V: C104.1 C106.1 IC101.3 POWER.5 Q101.D2 Q101.D2' Q102.D2 Q102.D2' R2.1
GND: C1.2 C2.2 C101.- C102.- C103.2 C104.2 C105.2 C106.2 C114.2 C201.2 C202.2 C301.2 C302.1 C303.2 C401.2 C402.2 C403.2 C503.2 C504.2 C505.2 C506.2 C601.2 C602.2 C603.2 C701.1 C801.2 C802.2 C803.2 C804.2 C805.2 C806.2 C807.2 C808.1 C809.1 C810.2 C811.1 C901.2 C902.1 C903.2 C904.2 C905.2 C906.1 C907.1 GND800.X IC1.3 IC2.3 IC101.1 IC105.3 IC105.12 IC105.13 IC105.14 IOH.7 J201.-1 J201.-2 J201.-3 J201.E1 J201.E2 J201.E3 PB901.1 PB901.2 PB901.5 POWER.6 POWER.7 Q105.1 Q105.4 Q301.1 Q301.4 R1.2 R101.2 R124.1 R129.1 R131.1 R302.2 R305.1 R306.1 R307.1 R308.2 R801.1 R810.1 SPI1.6 U201.2 U201.3 U201.6 U201.7 U301.6 U301.12 U301.14 U301.26 U301.30 U301.GND@1 U301.GND@2 U301.GND@3 U301.GND@4 U301.GND@5 U301.GND@6 U301.GND@7 U301.GND@8 U301.GND@9 U301.GND@10 U301.GND@11 U301.GND@12 U401.P$2 U502.2 U502.11 U502.12 U502.13 U502.14 U502.15 U502.16 U502.22 U504.3 U504.4 U504.7 U504.11 U504.12 U504.13 U504.22 U601.P$2 U701.4 U701.9 U801.5 U801.15 U801.23 U801.35 U801.43 U801.45 U901.15 U901.29 U901.43 USB801.GND X801.2 X801.4
MEDBG1:N$1: C801.1 D801.1 R801.2 USB801.SHIELD1 USB801.SHIELD2
MEDBG1:N$2: F801.2 USB801.VBUS
MEDBG1:N$3: C802.1 F801.1 L801.1
MEDBG1:N$4: R802.1 U801.1
MEDBG1:N$5: C804.1 U801.6
MEDBG1:N$6: C805.1 R803.1 RST800.X U801.13
MEDBG1:N$7: C811.2 U801.16 X801.1
MEDBG1:N$8: C810.1 U801.17 X801.3
MEDBG1:N$9: R804.2 U801.20
MEDBG1:N$10: R805.2 U801.21
MEDBG1:N$11: LTX800.C U801.27
MEDBG1:N$12: R806.1 U801.25
MEDBG1:N$13: LRX800.C U801.26
MEDBG1:N$14: LTX800.A R808.1
MEDBG1:N$15: LRX800.A R807.1
MEDBG1:N$16: R809.1 R810.2 TP801.X U801.33
MEDBG1:N$17: MISO800.X U801.11
MEDBG1:N$18: MOSI800.X U801.10
MEDBG1:N$19: SCK800.X U801.9
MEDBG1:USB2_N: R811.1 U801.3
MEDBG1:USB2_PI: R812.1 U801.4
MEDBG1:USB_N: D801.3 R811.2 USB801.D-
MEDBG1:USB_P: D801.2 R812.2 USB801.D+
N$1: U301.20 U401.P$5
N$2: U301.1 U502.18
N$3: U301.22 U502.19
N$4: U201.14 U301.36 U504.19
N$5: U301.23 U504.18
N$6: U201.1 U502.20
N$7: U301.27 U401.P$4
N$8: U301.28 U504.16
N$9: IC1.2 U502.6
N$10: IC2.2 U502.4
N$12: R304.2 U601.P$5
N$13: R303.2 U601.P$4
N$14: JP1.1 R4.2 R802.2 R901.1 U901.41
N$15: U201.4 U502.21
N$16: U201.12 U504.14
N$17: R903.2 U801.29
N$18: U301.7 U502.17
N$19: R805.1 U901.9
N$20: R804.1 U901.8
N$21: U901.26 USR.A
N$22: R1.1 USR.C
N$23: U201.13 U301.29 U504.15
PA0: IOL.3 U901.44
PA1: IOL.8 U901.45
PA2: IOH.9 U601.P$1 U701.5 U901.46
PA3: IOH.10 U601.P$8 U701.6 U901.47
PA4: U504.6 U901.48
PA5: U502.5 U901.1
PA6: U401.P$1 U901.2
PA7: Q301.2 R302.1 U901.3
PB0: IOH.2 U901.4
PB1: IOH.3 U901.5
PB2: IOL.6 U901.6
PB3: IC2.1 R5.1 U504.10 U901.7
PC0: SPI1.4 U504.5 U901.10
PC1: IC1.4 IC2.4 SPI1.1 U901.11
PC2: SPI1.3 U504.9 U901.12
PC3: U901.13
PC4: IOL.2 U901.16
PC5: IOL.1 U901.17
PC6: IOL.5 U901.18
PC7: U502.3 U901.19
PD0: AD.1 U901.20
PD1: AD.2 U901.21
PD2: AD.3 U901.22
PD3: AD.4 U901.23
PD4: AD.5 U901.24
PD5: AD.6 U901.25
PD7: C1.1 C2.1 IOH.8 U901.27
PE0: IOH.4 U901.30
PE1: IOH.5 U901.31
PE2: IOH.6 U901.32
PE3: IOH.1 U901.33
PF2: IC1.1 R11.1 U504.8 U901.36
PF3: U502.7 U901.37
PF4: IOL.7 U901.38
PF5: IOL.4 U901.39
PWR1:N17690335: Q101.S1 Q101.S2 R127.2
PWR1:N17690346: Q101.G1 Q101.G2 Q105.6 R127.1
PWR1:N17690381: Q105.2 R125.1 R126.2
PWR1:N17690821: Q102.S1 Q102.S2 R128.2
PWR1:N17690840: Q102.G1 Q102.G2 Q105.3 R126.1 R128.1
PWR1:N17690878: C114.1 Q105.5 R123.1 R124.2
PWR1:N$1: D101.A J201.+1 J201.+2 J201.+3
PWR1:N$3: C102.+ C103.1 IC105.7 IC105.8 IC105.9 IC105.20 Q102.D1 Q102.D1' R102.2 R123.2
PWR1:N$4: ON100.C R101.1
PWR1:N$35: IC105.1 R102.1 R129.2
PWR1:N$36: IC105.17 R130.2
PWR1:N$37: IC105.18 R131.2
TRG_RST: C903.1 POWER.3 Q301.3 R806.2 R902.1 R903.1 R904.1 SPI1.5 U901.40
UC1:N$2: PB901.3 PB901.4 R904.2
UC1:N$3: C905.1 U901.34 Y901.1
UC1:N$4: C904.1 U901.35 Y901.2
UPDI_REMOTE: R4.1 U401.P$8
VDD: C403.1 C503.1 C504.1 C603.1 C701.2 C806.1 C807.1 C808.2 C809.2 C901.1 C902.2 C906.2 C907.2 IC1.5 IC2.5 POWER.2 R2.2 R3.2 R5.2 R11.2 R504.2 R803.2 R807.2 R808.2 R809.2 R901.2 R902.2 SPI1.2 U401.P$7 U502.1 U504.1 U601.P$7 U701.8 U801.2 U801.14 U801.24 U801.34 U801.42 U801.44 U901.14 U901.28 U901.42 VDD800.X
VIN: C101.+ D101.C IC105.16 POWER.8 R130.1
VUSB: C803.1 D801.4 L801.2 Q101.D1 Q101.D1' R125.2 U801.7
WIFI/BLE1:N$1: C303.1 Q301.6 R301.1 U301.19
WIFI/BLE1:N$2: R303.1 U301.35
WIFI/BLE1:N$3: R304.1 U301.31
WIFI/BLE1:N$4: DL301.2 U301.16
WIFI/BLE1:N$5: DL301.1 U301.17
WIFI/BLE1:N$6: DL301.3 U301.18
WIFI/BLE1:N$7: DL301.5 R305.2
WIFI/BLE1:N$8: DL301.6 R306.2
WIFI/BLE1:N$9: DL301.4 R307.2
WIFI/BLE1:N$10: R309.2 U301.24
WIFI/BLE1:N$11: Q301.5 R308.1 R309.1 R310.1
WIFI/BLE1:N$12: R310.2 U301.21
